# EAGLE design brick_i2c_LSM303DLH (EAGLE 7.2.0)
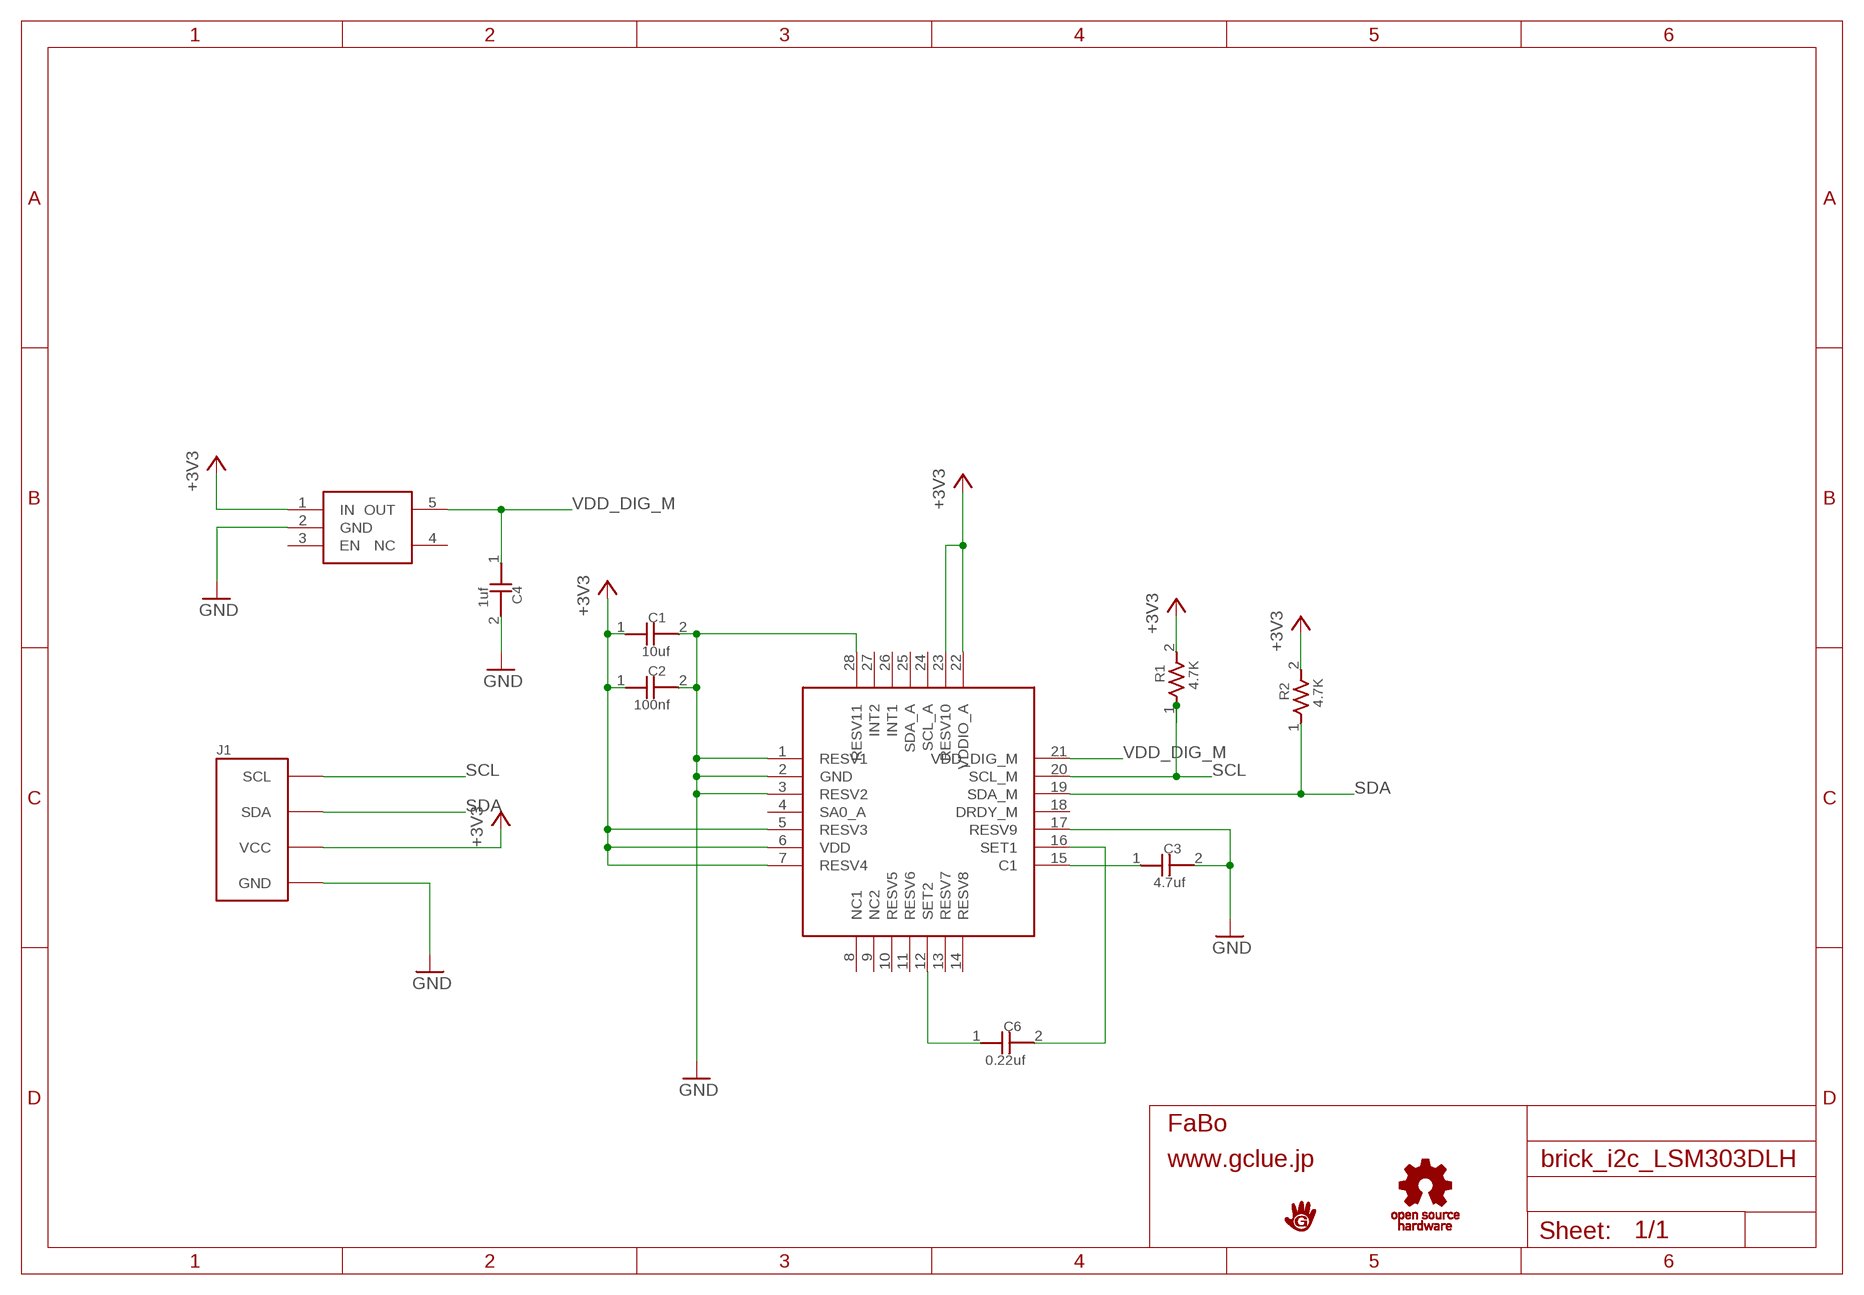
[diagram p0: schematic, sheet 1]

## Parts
C1  10uf  CAPACITOR0603  [0603]
C2  100nf  CAPACITOR0603  [0603]
C3  4.7uf  CAPACITOR0603  [0603]
C4  1uf  CAPACITOR0603  [0603]
C6  0.22uf  CAPACITOR0603  [0603]
J1  BRICK_I2C  [BRICK_I2C]
R1  4.7K  RESISTOR0603  [0603]
R2  4.7K  RESISTOR0603  [0603]
U$2  ST-LSM303DLH  [LGA-28]
U$3  TI-TLV70018DDCT  [SOT23-5]
U$4  LOGO_GCLUE-M  [LOGO_GCLUE_M]
U$5  LOGO_OSHW_T-M  [LOGO_OSHW_T_M]

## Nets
+3V3: C1.1 C2.1 J1.VCC R1.2 R2.2 U$2.5(RESV3) U$2.6(VDD) U$2.7(RESV4) U$2.22(VDDIO_A) U$2.23(RESV10) U$3.1(IN)
GND: C1.2 C2.2 C3.2 C4.2 J1.GND U$2.1(RESV1) U$2.2(GND) U$2.3(RESV2) U$2.17(RESV9) U$2.28(RESV11) U$3.2(GND)
N$1: C6.1 U$2.12(SET2)
N$2: C6.2 U$2.16(SET1)
N$3: C3.1 U$2.15(C1)
SCL: J1.SCL R1.1 U$2.20(SCL_M)
SDA: J1.SDA R2.1 U$2.19(SDA_M)
VDD_DIG_M: C4.1 U$2.21(VDD_DIG_M) U$3.5(OUT)
Unconnected: U$2.4(SA0_A) U$2.8(NC1) U$2.9(NC2) U$2.10(RESV5) U$2.11(RESV6) U$2.13(RESV7) U$2.14(RESV8) U$2.18(DRDY_M) U$2.24(SCL_A) U$2.25(SDA_A) U$2.26(INT1) U$2.27(INT2) U$3.3(EN) U$3.4(NC)

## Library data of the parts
C1-C4 C6 = GClue-Capacitor:CAPACITOR
J1 = gclue:BRICK_I2C: FaBo Brick 4pin(I2C)
R1 R2 = GClue-Resistors:RESISTOR
U$2 = GClue-Mems:ST-LSM303DLH
U$3 = gclueParts:TI-TLV70018DDCT
U$4 = gclue:LOGO_GCLUE
U$5 = gclue:LOGO_OSHW_T

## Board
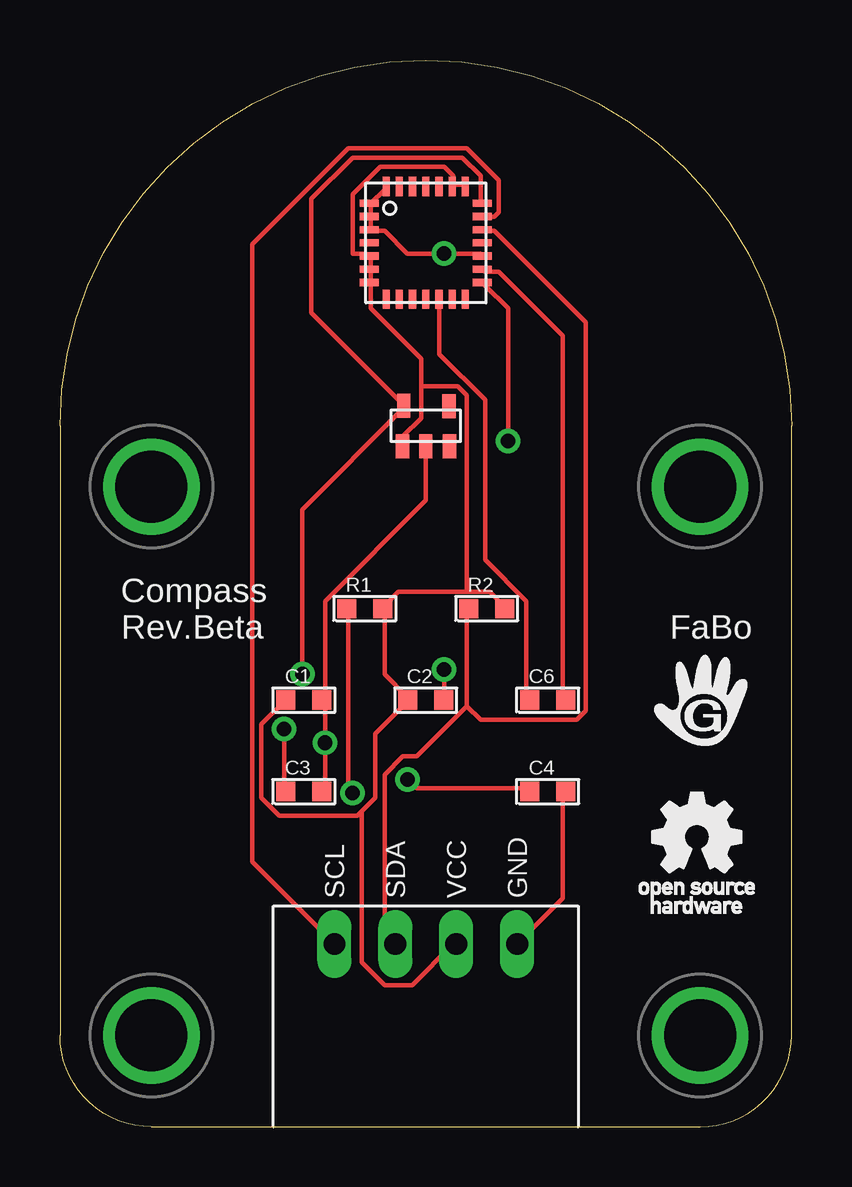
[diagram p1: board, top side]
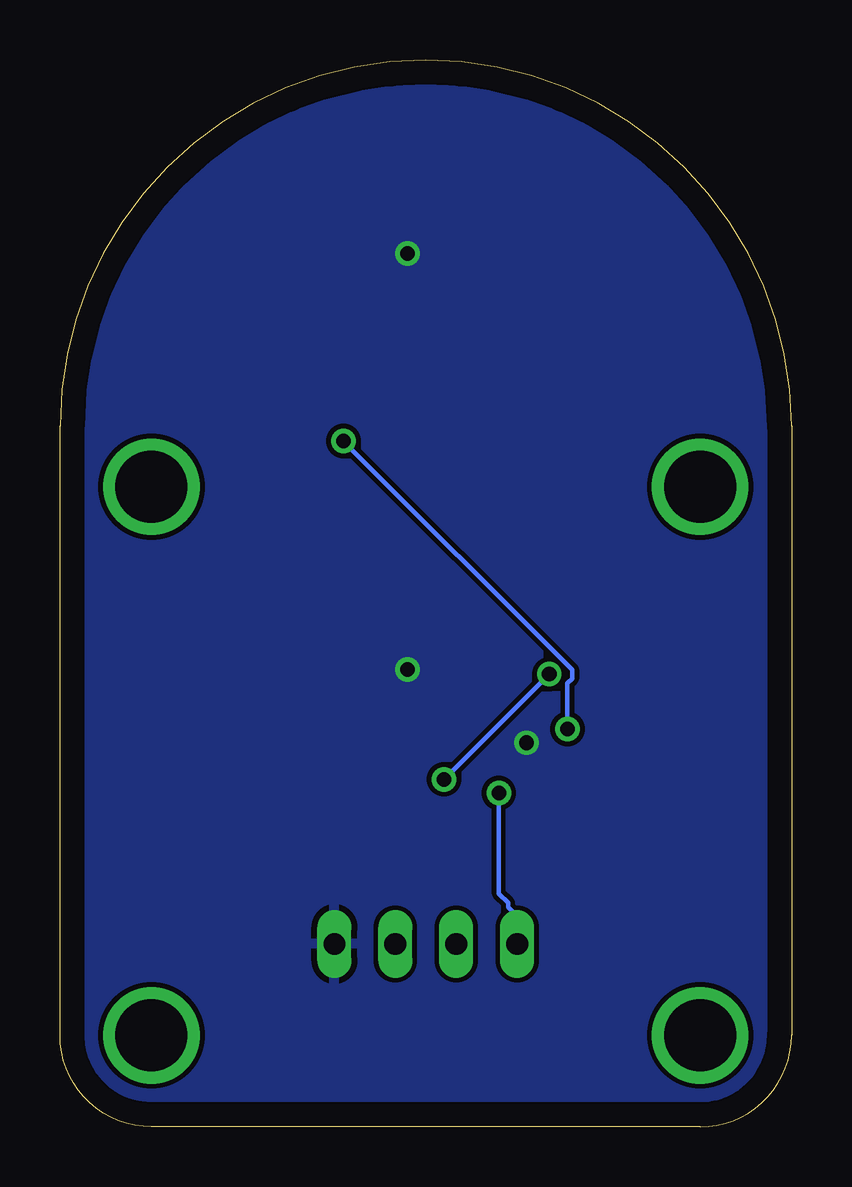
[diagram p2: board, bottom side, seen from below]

Size 30.48 x 44.45 mm. Coordinates in mm from the lower left corner, seen from the top.
Copper layers (1*16): Top 0.035mm / dielectric 1.5mm / Bottom 0.035mm
Design rules "default *": minimum track width 7mil, minimum drill 24mil, track to track 8mil, track to pad 8mil, pad to pad 8mil, via to via 8mil, smd to smd 8mil, copper to edge 40mil, drill to drill 8mil, minimum pad ring 10mil, minimum via ring 8mil, stop-mask expansion 4mil, vias tented up to drill 0mil, thermal gap 10mil

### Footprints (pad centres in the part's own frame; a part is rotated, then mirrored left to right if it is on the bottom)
0603 = smd 0.8 x 0.8: 1 -0.75,0; 2 0.75,0
BRICK_I2C = drill 0.9 long: GND 3.81,-11.43; SCL -3.81,-11.43; SDA -1.27,-11.43; VCC 1.27,-11.43 | drill 3 pad 3.81: P$5 -11.43,7.62; P$6 11.43,7.62; P$7 -11.43,-15.24; P$8 11.43,-15.24
LGA-28 = smd 0.8 x 0.3: 1 -2.35,1.65; 2 -2.35,1.1; 3 -2.35,0.55; 4 -2.35,0; 5 -2.35,-0.55; 6 -2.35,-1.1; 7 -2.35,-1.65; 15 2.35,-1.65; 16 2.35,-1.1; 17 2.35,-0.55; 18 2.35,0; 19 2.35,0.55; 20 2.35,1.1; 21 2.35,1.65 | smd 0.3 x 0.8: 8 -1.65,-2.35; 9 -1.1,-2.35; 10 -0.55,-2.35; 11 0,-2.35; 12 0.55,-2.35; 13 1.1,-2.35; 14 1.65,-2.35; 22 1.65,2.35; 23 1.1,2.35; 24 0.55,2.35; 25 0,2.35; 26 -0.55,2.35; 27 -1.1,2.35; 28 -1.65,2.35
SOT23-5 = smd 0.55 x 1: 1 -0.97,-0.85; 2 0,-0.85; 3 0.99,-0.85; 4 0.97,0.82; 5 -0.92,0.84

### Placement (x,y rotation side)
C1  10.16,17.78 0 top
C2  15.24,17.78 0 top
C3  10.16,13.97 0 top
C4  20.32,13.97 0 top
C6  20.32,17.78 0 top
J1  15.24,19.05 0 top
R1  12.7,21.59 0 top
R2  17.78,21.59 0 top
U$2  15.24,36.83 0 top
U$3  15.24,29.21 0 top
U$4  26.67,17.78 0 top
U$5  26.67,11.43 0 top

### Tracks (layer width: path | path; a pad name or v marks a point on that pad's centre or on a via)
+3V3
  Top 0.178: 16.38,39.24 16.76,39.24 U$2.22 | 16.38,39.24 16.38,39.62 16,40.01 13.34,40.01 12.19,38.86 12.19,36.39 12.76,36.39 U$2.5 12.95,36.2 12.95,35.81 U$2.6 12.95,35.62 12.95,35.24 U$2.7 12.95,35.05 12.95,34.1 15.05,32 15.05,30.86 | 16.38,39.24 U$2.23 | 15.05,30.86 15.05,29.53 14.29,28.77 14.29,28.38 U$3.1 | 12.57,13.14 13.14,13.72 13.14,16.38 14.48,17.72 C2.1 14.48,17.91 13.53,18.86 13.53,21.53 R1.2 13.53,21.72 14.1,22.29 16.95,22.29 | 12.57,13.14 12.38,12.95 9.14,12.95 8.38,13.72 8.38,16.76 9.34,17.72 C1.1 | 16.95,22.29 17.91,22.29 18.48,21.72 R2.2 | 12.57,13.14 12.57,6.86 13.53,5.91 14.67,5.91 16.38,7.62 J1.VCC | 15.05,30.86 16.57,30.86 16.95,30.48 16.95,22.29
GND  (via drill 0.61)
  Top 0.178: C3.2 11.05,14.1 v11.05,16 11.05,17.72 C1.2 11.05,17.91 11.05,21.91 15.24,26.1 U$3.2 | 12.95,37.91 12.95,37.53 U$2.3 12.95,37.34 13.53,37.34 14.48,36.39 v16,36.39 17.53,36.39 U$2.17 | 12.95,37.91 12.95,38.48 | 12.95,37.91 U$2.2 | 12.95,38.48 13.53,39.05 U$2.28 | 12.95,38.48 U$2.1 | J1.GND 20.95,9.53 20.95,13.91 C4.2 | v16,19.05 16,17.91 C2.2
  pour Bottom: 0,0 30.48,0 30.48,44.45 0,44.45
N$1
  Top 0.178: U$2.12 15.81,34.29 15.81,32.19 17.72,30.29 17.72,23.62 19.43,21.91 19.43,17.91 C6.1
N$2
  Top 0.178: U$2.16 17.72,35.62 18.29,35.62 20.95,32.96 20.95,17.91 C6.2
N$3  (via drill 0.61)
  Top 0.178: v9.34,16.57 9.34,14.1 C3.1 | v18.67,28.57 18.67,34.1 17.72,35.05 U$2.15
  Bottom 0.178: v9.34,16.57 9.34,18.48 9.14,18.67 9.14,19.05 v18.67,28.57
SCL  (via drill 0.61)
  Top 0.178: v12.19,13.91 12,14.1 12,21.53 R1.1 | J1.SCL 8,11.05 8,36.77 12,40.77 16.95,40.77 18.29,39.43 18.29,38.1 18.1,37.91 17.72,37.91 U$2.20
  Bottom 0.178: v12.19,13.91 12.19,9.72 11.81,9.34 11.81,9.14 11.43,8.76 J1.SCL
SDA
  Top 0.178: 16.95,17.53 16.95,21.53 R2.1 | 16.95,17.53 14.86,15.43 14.29,15.43 13.53,14.67 13.53,8 13.91,7.62 J1.SDA | 16.95,17.53 17.53,16.95 21.53,16.95 21.91,17.34 21.91,33.53 18.1,37.34 17.72,37.34 U$2.19
VDD_DIG_M  (via drill 0.61)
  Top 0.178: U$2.21 17.53,38.48 17.53,39.62 16.76,40.39 12.19,40.39 10.48,38.67 10.48,33.91 14.29,30.1 U$3.5 14.29,29.91 10.1,25.72 v10.1,18.86 | v14.48,14.48 14.86,14.1 19.43,14.1 C4.1
  Bottom 0.178: v10.1,18.86 v14.48,14.48

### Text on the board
tPlace: Compass / Rev.Beta | FaBo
